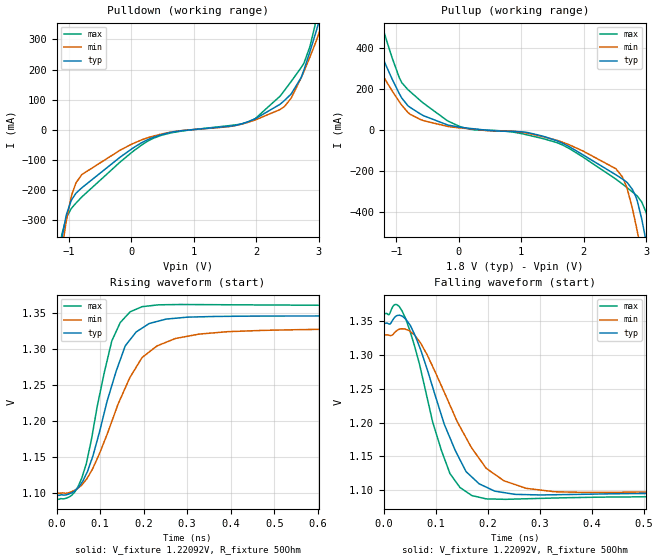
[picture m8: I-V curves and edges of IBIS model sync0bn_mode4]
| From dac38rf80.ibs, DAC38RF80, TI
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|   sync0bn_mode4 Model
[Model]   sync0bn_mode4
Model_type   Output
Polarity   Non-Inverting
Vmeas = 1.220921
Vref = 1.220921
Cref = 2pF
Rref = 200
|   typ   min   max
|   (nom PVT)   (fast PVT)   (slow PVT)
C_comp   6.001e-13   5.910e-13   7.162e-13
| Where nom  PVT is Nominal Process, 1.8V, 27C
|   Fast PVT is Strong Process,  1.89V, -40C
|   Slow PVT is Weak Process,   1.71V, 105C
[Voltage Range]   1.8   1.71   1.89
|Junction Temperature
[Temperature Range]   27   105   -40
[Pullup Reference]   1.8   1.71   1.89
[Pulldown Reference]   0   0   0
[Power Clamp Reference]   1.8   1.71   1.89
[GND Clamp Reference]   0   0   0
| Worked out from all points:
|   slope of the pulldown table from 0 to 0.27 V, typ, clamps not added: 8.4 ohm
|   slope of the pullup table from 0 to 0.27 V, typ, clamps not added: 28.8 ohm
|   falling waveform, V_fixture 1.22092V, R_fixture 50Ohm: 20-80 % time 69.7ps typ, 91ps min, 56.1ps max; typ from 1.35 V to 1.1 V
|   rising waveform, V_fixture 1.22092V, R_fixture 50Ohm: 20-80 % time 71.9ps typ, 99.2ps min, 54.9ps max; typ from 1.1 V to 1.35 V
[Pulldown]
|   Voltage   I(typ)   I(min)   I(max)
-1.8V     -1.51A     -1.417A    -1.67A
-1.112V   -358.5mA   -395.5mA   -346.1mA
-968.9mV  -237.8mA   -226.6mA   -263.4mA
-796.2mV  -193.2mA   -149.1mA   -223.6mA
1.17mV    -64.1mA    -48.19mA   -75.91mA
510.2mV   -14.67mA   -12.96mA   -16.78mA
1.861V    26.15mA    24.33mA    25.34mA
2.381V    84.81mA    67.26mA    111.9mA
2.716V    172.8mA    171.9mA    206.3mA
2.965V    332mA      298.3mA    371.7mA
3.086V    417.6mA    369mA      505.2mA
3.6V      891.3mA    1.263A     1.165A
[Pullup]
|   Voltage   I(typ)   I(min)   I(max)
-1.8V     837.7mA    987.5mA    1.203A
-1.6V     623.8mA    537mA      949.4mA
-1.427V   497.2mA    379.3mA    732.4mA
-1.302V   408.1mA    309.3mA    583.5mA
-783.2mV  109.5mA    76.07mA    186.6mA
36mV      11.42mA    8.128mA    13.83mA
1.791V    -86.51mA   -76.53mA   -95.51mA
2.619V    -239.5mA   -229.5mA   -264.1mA
2.859V    -348.2mA   -496.2mA   -323.4mA
2.992V    -531.9mA   -691.9mA   -396.8mA
3.069V    -662.7mA   -806.3mA   -489.4mA
3.6V      -1.567A    -1.599A    -1.551A
[Ramp]
R_load = 50
|   typ   min   max
dV/dt_r   0.14958/7.1826e-11   0.13776/9.6e-11   0.120054/8.33008e-11
dV/dt_f   0.149616/6.97281e-11   0.137422/9.09244e-11   0.16142/5.60533e-11
[Falling Waveform]
V_fixture = 1.22092V
V_fixture_min = 1.21354V
V_fixture_max = 1.22548V
R_fixture = 50Ohm
|   Time   V(typ)   V(min)   V(max)
0s        1.346V     1.329V     1.36V
24.83ps   1.358V     1.336V     1.374V
51.03ps   1.343V     1.334V     1.333V
93.6ps    1.252V     1.283V     1.201V
126.9ps   1.178V     1.226V     1.125V
157.8ps   1.128V     1.178V     1.098V
196.6ps   1.105V     1.133V     1.088V
234.1ps   1.096V     1.113V     1.087V
327.9ps   1.094V     1.098V     1.089V
1.699ns   1.097V     1.1V       1.091V
[Rising Waveform]
V_fixture = 1.22092V
V_fixture_min = 1.21354V
V_fixture_max = 1.22548V
R_fixture = 50Ohm
|   Time   V(typ)   V(min)   V(max)
0s        1.097V     1.1V       1.091V
34.9ps    1.1V       1.102V     1.097V
60.34ps   1.116V     1.113V     1.125V
83.72ps   1.152V     1.135V     1.187V
126.9ps   1.249V     1.199V     1.312V
157.8ps   1.305V     1.246V     1.345V
196.6ps   1.33V      1.289V     1.359V
273.3ps   1.343V     1.315V     1.362V
393.5ps   1.346V     1.325V     1.362V
1.699ns   1.346V     1.329V     1.36V
